FUNCTION_BLOCK "FB_CABINET_7P7-R24"
TITLE =Control cabinet 7P7-R24
{ S7_language := '9(1) Angielski (Stany Zjednoczone)  11.01.2022  09:45:15' }
VERSION : 0.1


VAR
  SM : STRUCT
   GeneralError : BOOL ;
   GeneralWarning : BOOL ;
   CtrlVoltageON : BOOL ;
   Auto : BOOL ;
   Manual : BOOL ;
   Local : BOOL ;
   Remote : BOOL ;
   CtrlRelease : BOOL ;
   CtrlRelease_A : BOOL ;
   res11 : BOOL ;
   res12 : BOOL ;
   res13 : BOOL ;
   res14 : BOOL ;
   res15 : BOOL ;
   LackCooling : BOOL ;
   LackHeating : BOOL ;
  END_STRUCT ;
  FM : STRUCT
   EnergyCounterFuse : BOOL ;
   ControlVoltage230VAC : BOOL ;
   ControlVoltage24VDC : BOOL ;
   ControlVoltage230VAC_MS : BOOL ;
   CabinetCoolingFuse : BOOL ;
   ProfiNetSwitchFault : BOOL ;
   MainSwitchFault : BOOL ;
   ExcessTemperature : BOOL ;
   ESTOP : BOOL ;
   FireAlarmPreWarning : BOOL ;
   FireAlarm : BOOL ;
   res13 : BOOL ;
   res14 : BOOL ;
   res15 : BOOL ;
   res16 : BOOL ;
   res17 : BOOL ;
  END_STRUCT ;
  CTRL : STRUCT
   ResetFault : BOOL ;
   ResetESTOP : BOOL ;
   LampTest : BOOL ;
   AutoStart : BOOL ;
   AutoStop : BOOL ;
   res05 : BOOL ;
   res06 : BOOL ;
   res07 : BOOL ;
   res10 : BOOL ;
   res11 : BOOL ;
   res12 : BOOL ;
   res13 : BOOL ;
   res14 : BOOL ;
   res15 : BOOL ;
   res16 : BOOL ;
   res17 : BOOL ;
  END_STRUCT ;
  CTRL_HMI : STRUCT
   ResetFault : BOOL ;
   Auto : BOOL ;
   Manual : BOOL ;
   res03 : BOOL ;
   res04 : BOOL ;
   res05 : BOOL ;
   res06 : BOOL ;
   res07 : BOOL ;
   ProductionOn : BOOL ;
   ProductionBreak : BOOL ;
   PlantOn : BOOL ;
   PlantOff : BOOL ;
   res14 : BOOL ;
   res15 : BOOL ;
   LackCooling : BOOL ;
   LackHeating : BOOL ;
  END_STRUCT ;
  EC : "UDT_EC";	//Energy Counter
END_VAR
VAR_TEMP
  ERROR_REL : BOOL ;
END_VAR
BEGIN
NETWORK
TITLE =STATUS



NETWORK
TITLE =CONTROL VOLTAGE ON
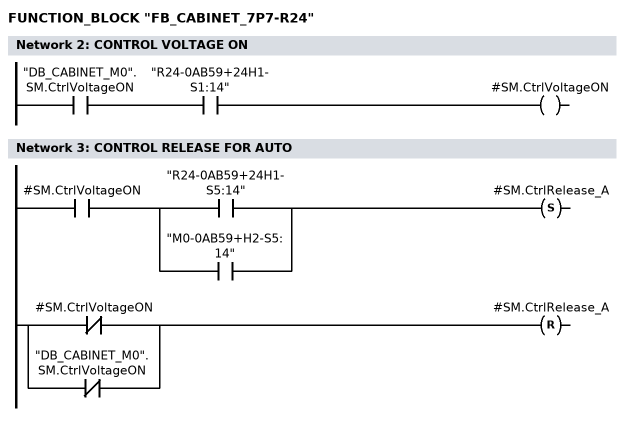
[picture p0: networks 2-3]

      U     "DB_CABINET_M0".SM.CtrlVoltageON;
      U     "R24-0AB59+24H1-S1:14";
      =     #SM.CtrlVoltageON;
NETWORK
TITLE =CONTROL RELEASE FOR AUTO

      U     #SM.CtrlVoltageON;
      U(    ;
      O     "R24-0AB59+24H1-S5:14";
      O     "M0-0AB59+H2-S5:14";
      )     ;
      S     #SM.CtrlRelease_A;
      U(    ;
      ON    #SM.CtrlVoltageON;
      ON    "DB_CABINET_M0".SM.CtrlVoltageON;
      )     ;
      R     #SM.CtrlRelease_A;
      NOP   0;
NETWORK
TITLE =AUTO/MANUAL MODE

      U(    ;
      U     "R24-0AB59+24H1-S2:14";
      S     #SM.Auto;
      U     "R24-0AB59+24H1-S2:22";
      R     #SM.Auto;
      U     #SM.Auto;
      )     ;
      NOT   ;
      =     #SM.Manual;
NETWORK
TITLE =LOCAL/REMOTE MODE

      U(    ;
      U     "DB_CABINET_M0".SM.Remote;
      S     #SM.Remote;
      U     "DB_CABINET_M0".SM.Local;
      R     #SM.Remote;
      U     #SM.Remote;
      )     ;
      NOT   ;
      =     #SM.Local;
NETWORK
TITLE =CONTROL RELEASE FROM CABINET
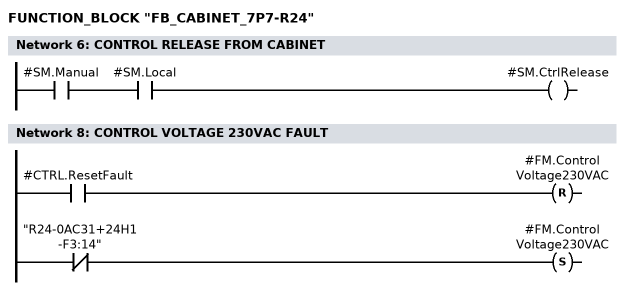
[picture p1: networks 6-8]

      U     #SM.Manual;
      U     #SM.Local;
      =     #SM.CtrlRelease;
NETWORK
TITLE =FAULTS



NETWORK
TITLE =CONTROL VOLTAGE 230VAC FAULT

      U     #CTRL.ResetFault;
      R     #FM.ControlVoltage230VAC;
      UN    "R24-0AC31+24H1-F3:14";
      S     #FM.ControlVoltage230VAC;
      NOP   0;
NETWORK
TITLE =CONTROL VOLTAGE 24V DC FAULT

      U     #CTRL.ResetFault;
      R     #FM.ControlVoltage24VDC;
      U(    ;
      O(    ;
      UN    "R24-0DC43+24H1-F1:7";
      L     S5T#300MS;
      SE    "T_R24-0DC43+24H1-F1";
      NOP   0;
      NOP   0;
      NOP   0;
      U     "T_R24-0DC43+24H1-F1";
      )     ;
      O(    ;
      UN    "R24-0DC43+24H1-F2:7";
      L     S5T#300MS;
      SE    "T_R24-0DC43+24H1-F2";
      NOP   0;
      NOP   0;
      NOP   0;
      U     "T_R24-0DC43+24H1-F2";
      )     ;
      )     ;
      S     #FM.ControlVoltage24VDC;
      NOP   0;
NETWORK
TITLE =CONTROL VOLTAGE 230V AC BEFORE MAIN SWITCH FAULT
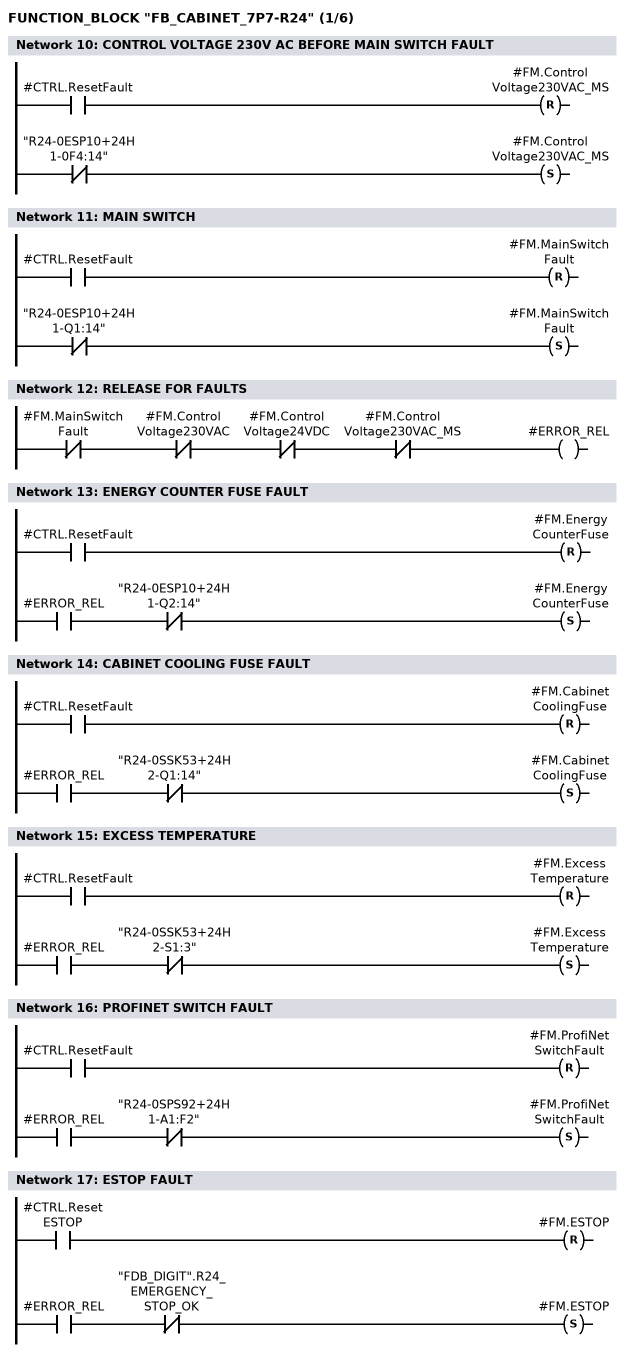
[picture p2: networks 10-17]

      U     #CTRL.ResetFault;
      R     #FM.ControlVoltage230VAC_MS;
      UN    "R24-0ESP10+24H1-0F4:14";
      S     #FM.ControlVoltage230VAC_MS;
      NOP   0;
NETWORK
TITLE =MAIN SWITCH

      U     #CTRL.ResetFault;
      R     #FM.MainSwitchFault;
      UN    "R24-0ESP10+24H1-Q1:14";
      S     #FM.MainSwitchFault;
      NOP   0;
NETWORK
TITLE =RELEASE FOR FAULTS

      UN    #FM.MainSwitchFault;
      UN    #FM.ControlVoltage230VAC;
      UN    #FM.ControlVoltage24VDC;
      UN    #FM.ControlVoltage230VAC_MS;
      =     #ERROR_REL;
NETWORK
TITLE =ENERGY COUNTER FUSE FAULT

      U     #CTRL.ResetFault;
      R     #FM.EnergyCounterFuse;
      U     #ERROR_REL;
      UN    "R24-0ESP10+24H1-Q2:14";
      S     #FM.EnergyCounterFuse;
      NOP   0;
NETWORK
TITLE =CABINET COOLING FUSE FAULT

      U     #CTRL.ResetFault;
      R     #FM.CabinetCoolingFuse;
      U     #ERROR_REL;
      UN    "R24-0SSK53+24H2-Q1:14";
      S     #FM.CabinetCoolingFuse;
      NOP   0;
NETWORK
TITLE =EXCESS TEMPERATURE

      U     #CTRL.ResetFault;
      R     #FM.ExcessTemperature;
      U     #ERROR_REL;
      UN    "R24-0SSK53+24H2-S1:3";
      S     #FM.ExcessTemperature;
      NOP   0;
NETWORK
TITLE =PROFINET SWITCH FAULT

      U     #CTRL.ResetFault;
      R     #FM.ProfiNetSwitchFault;
      U     #ERROR_REL;
      UN    "R24-0SPS92+24H1-A1:F2";
      S     #FM.ProfiNetSwitchFault;
      NOP   0;
NETWORK
TITLE =ESTOP FAULT

      U     #CTRL.ResetESTOP;
      R     #FM.ESTOP;
      U     #ERROR_REL;
      UN    "FDB_DIGIT".R24_EMERGENCY_STOP_OK;
      S     #FM.ESTOP;
      NOP   0;
NETWORK
TITLE =ESTOP CONTROL CABINET OK
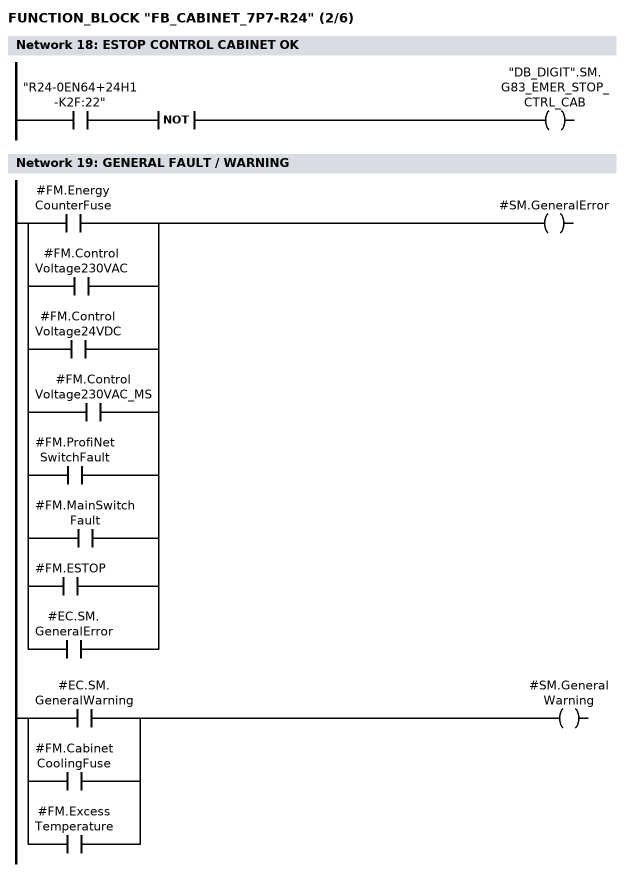
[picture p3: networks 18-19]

      U     "R24-0EN64+24H1-K2F:22";
      NOT   ;
      =     "DB_DIGIT".SM.G83_EMER_STOP_CTRL_CAB;
NETWORK
TITLE =GENERAL FAULT / WARNING


      U     #FM.EnergyCounterFuse;
      O     #FM.ControlVoltage230VAC;
      O     #FM.ControlVoltage24VDC;
      O     #FM.ControlVoltage230VAC_MS;
      O     #FM.ProfiNetSwitchFault;
      O     #FM.MainSwitchFault;
      O     #FM.ESTOP;
      O     #EC.SM.GeneralError;
      =     #SM.GeneralError;



      U     #EC.SM.GeneralWarning;
      O     #FM.CabinetCoolingFuse;
      O     #FM.ExcessTemperature;
      =     #SM.GeneralWarning;

NETWORK
TITLE =CONTROL SIGNALS



NETWORK
TITLE =RESET FAULT
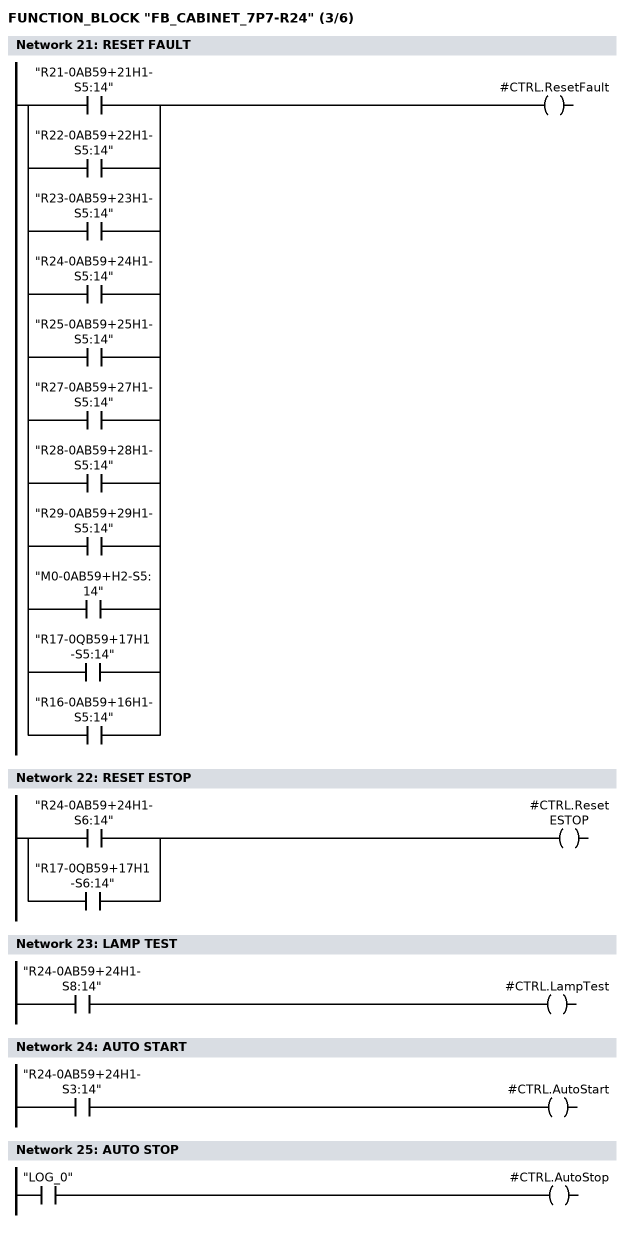
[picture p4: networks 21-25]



      O     "R21-0AB59+21H1-S5:14";
      O     "R22-0AB59+22H1-S5:14";
      O     "R23-0AB59+23H1-S5:14";
      O     "R24-0AB59+24H1-S5:14";
      O     "R25-0AB59+25H1-S5:14";
      O     "R27-0AB59+27H1-S5:14";
      O     "R28-0AB59+28H1-S5:14";
      O     "R29-0AB59+29H1-S5:14";
      O     "M0-0AB59+H2-S5:14";
      O     "R17-0QB59+17H1-S5:14";
      O     "R16-0AB59+16H1-S5:14";
      =     #CTRL.ResetFault;
NETWORK
TITLE =RESET ESTOP



      O     "R24-0AB59+24H1-S6:14";
      O     "R17-0QB59+17H1-S6:14";
      =     #CTRL.ResetESTOP;
NETWORK
TITLE =LAMP TEST



      U     "R24-0AB59+24H1-S8:14";
      =     #CTRL.LampTest;
NETWORK
TITLE =AUTO START



      U     "R24-0AB59+24H1-S3:14";
      =     #CTRL.AutoStart;
NETWORK
TITLE =AUTO STOP



      U     "LOG_0";
      =     #CTRL.AutoStop;
NETWORK
TITLE =BUTTON LAMPS
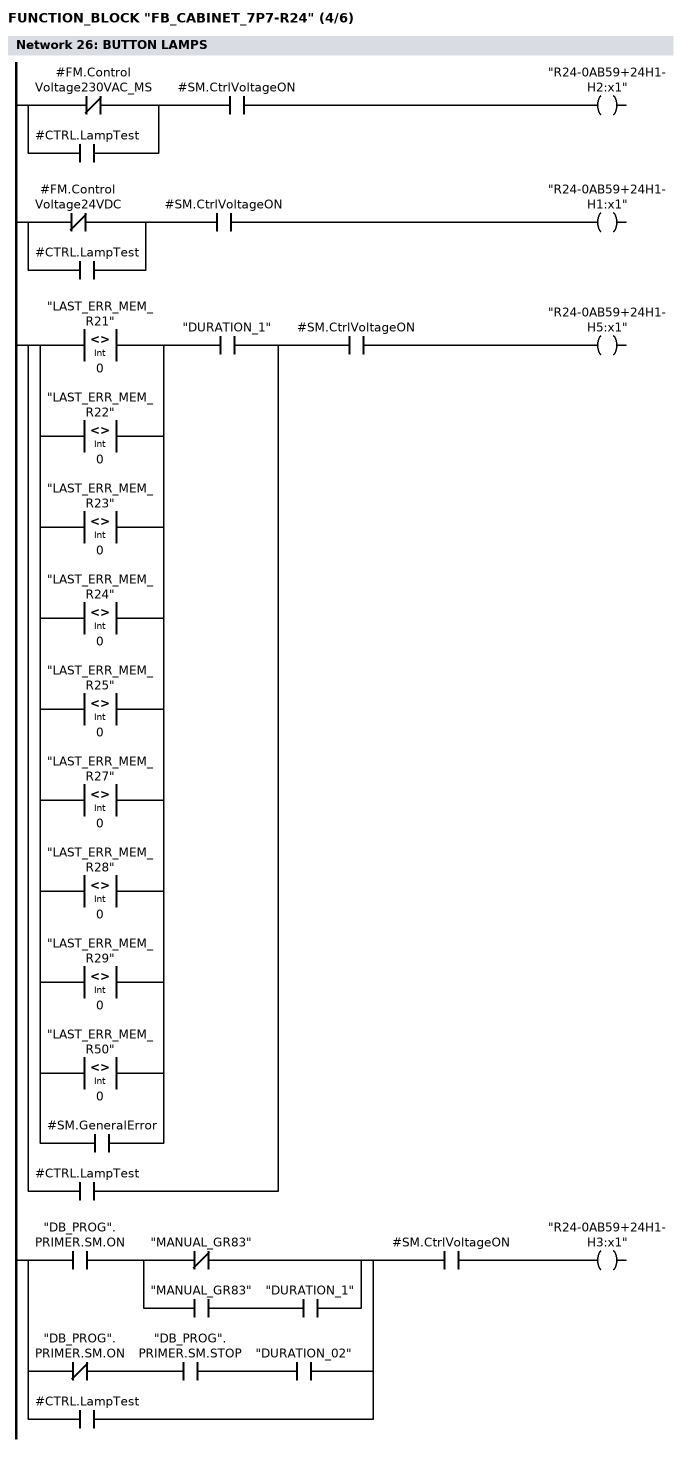
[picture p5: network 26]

// CONTROL VOLTAGE 230V AC
      U(    ;
      ON    #FM.ControlVoltage230VAC_MS;
      O     #CTRL.LampTest;
      )     ;
      U     #SM.CtrlVoltageON;
      =     "R24-0AB59+24H1-H2:x1";

// CONTROL VOLTAGE 24V DC
      U(    ;
      ON    #FM.ControlVoltage24VDC;
      O     #CTRL.LampTest;
      )     ;
      U     #SM.CtrlVoltageON;
      =     "R24-0AB59+24H1-H1:x1";

// RESET
      U(    ;
      L     "LAST_ERR_MEM_R21";
      L     0;
      <>I   ;
      )     ;
      O(    ;
      L     "LAST_ERR_MEM_R22";
      L     0;
      <>I   ;
      )     ;
      O(    ;
      L     "LAST_ERR_MEM_R23";
      L     0;
      <>I   ;
      )     ;
      O(    ;
      L     "LAST_ERR_MEM_R24";
      L     0;
      <>I   ;
      )     ;
      O(    ;
      L     "LAST_ERR_MEM_R25";
      L     0;
      <>I   ;
      )     ;
      O(    ;
      L     "LAST_ERR_MEM_R27";
      L     0;
      <>I   ;
      )     ;
      O(    ;
      L     "LAST_ERR_MEM_R28";
      L     0;
      <>I   ;
      )     ;
      O(    ;
      L     "LAST_ERR_MEM_R29";
      L     0;
      <>I   ;
      )     ;
      O(    ;
      L     "LAST_ERR_MEM_R50";
      L     0;
      <>I   ;
      )     ;
      O     #SM.GeneralError;
      U     "DURATION_1";
      O     #CTRL.LampTest;
      U     #SM.CtrlVoltageON;
      =     "R24-0AB59+24H1-H5:x1";

// AUTOMATIC START
      U(    ;
      U     "DB_PROG".PRIMER.SM.ON;
      U(    ;
      ON    "MANUAL_GR83";
      O     ;
      U     "MANUAL_GR83";
      U     "DURATION_1";
      )     ;
      O     ;
      UN    "DB_PROG".PRIMER.SM.ON;
      U     "DB_PROG".PRIMER.SM.STOP;
      U     "DURATION_02";
      O     #CTRL.LampTest;
      )     ;
      U     #SM.CtrlVoltageON;

      =     "R24-0AB59+24H1-H3:x1";
NETWORK
TITLE =LIGHT TOWER
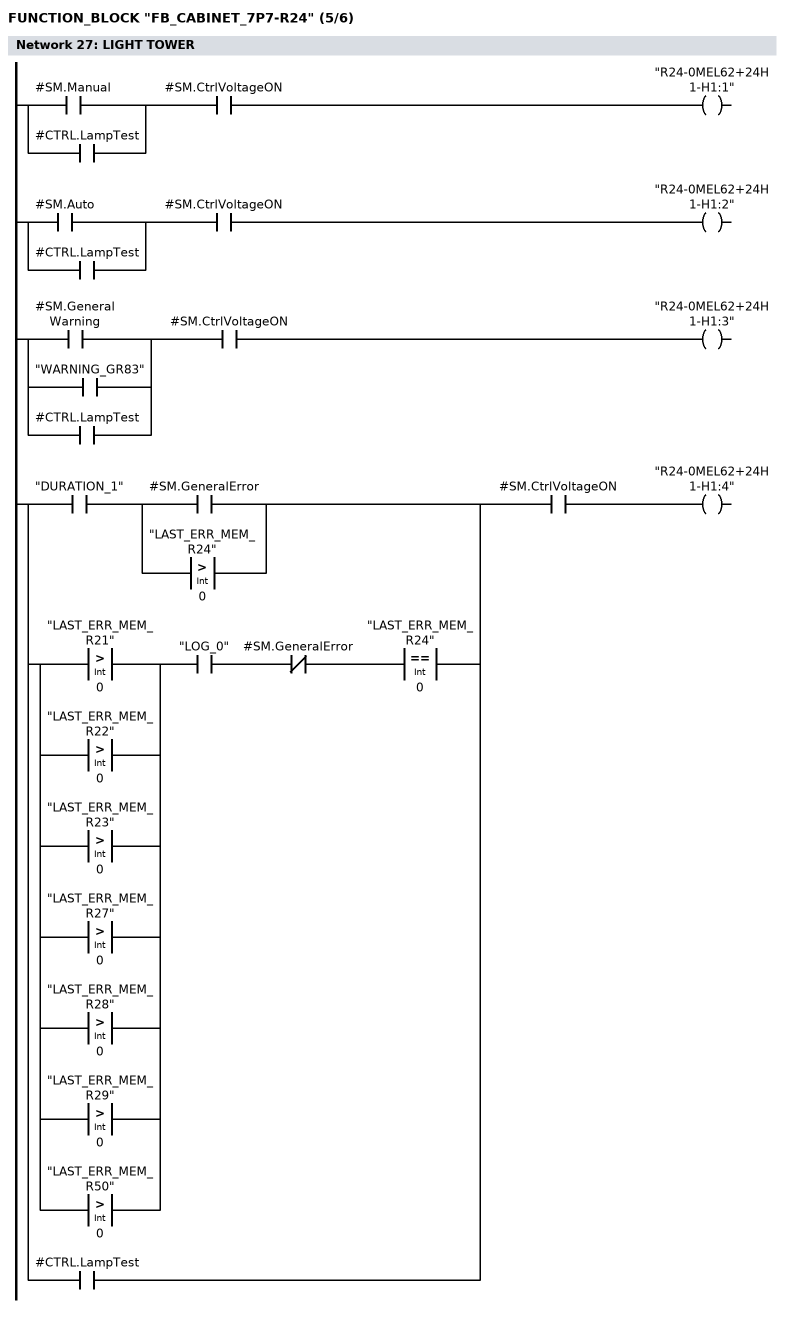
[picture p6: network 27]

// MANUAL
      U(    ;
      O     #SM.Manual;
      O     #CTRL.LampTest;
      )     ;
      U     #SM.CtrlVoltageON;
      =     "R24-0MEL62+24H1-H1:1";

// AUTO
      U(    ;
      O     #SM.Auto;
      O     #CTRL.LampTest;
      )     ;
      U     #SM.CtrlVoltageON;
      =     "R24-0MEL62+24H1-H1:2";

// WARNING
      U(    ;
      O     #SM.GeneralWarning;
      O     "WARNING_GR83";
      O     #CTRL.LampTest;
      )     ;
      U     #SM.CtrlVoltageON;
      =     "R24-0MEL62+24H1-H1:3";

// FAULT
      U(    ;
      U     "DURATION_1";
      U(    ;
      O     #SM.GeneralError;
      O(    ;
      L     "LAST_ERR_MEM_R24";
      L     0;
      >I    ;
      )     ;
      )     ;
      O     ;
      U(    ;
      O(    ;
      L     "LAST_ERR_MEM_R21";
      L     0;
      >I    ;
      )     ;
      O(    ;
      L     "LAST_ERR_MEM_R22";
      L     0;
      >I    ;
      )     ;
      O(    ;
      L     "LAST_ERR_MEM_R23";
      L     0;
      >I    ;
      )     ;
      O(    ;
      L     "LAST_ERR_MEM_R27";
      L     0;
      >I    ;
      )     ;
      O(    ;
      L     "LAST_ERR_MEM_R28";
      L     0;
      >I    ;
      )     ;
      O(    ;
      L     "LAST_ERR_MEM_R29";
      L     0;
      >I    ;
      )     ;
      O(    ;
      L     "LAST_ERR_MEM_R50";
      L     0;
      >I    ;
      )     ;
      )     ;
      U     "LOG_0";
      UN    #SM.GeneralError;
      U(    ;
      L     "LAST_ERR_MEM_R24";
      L     0;
      ==I   ;
      )     ;
      O     #CTRL.LampTest;
      )     ;
      U     #SM.CtrlVoltageON;
      =     "R24-0MEL62+24H1-H1:4";
NETWORK
TITLE =HORN
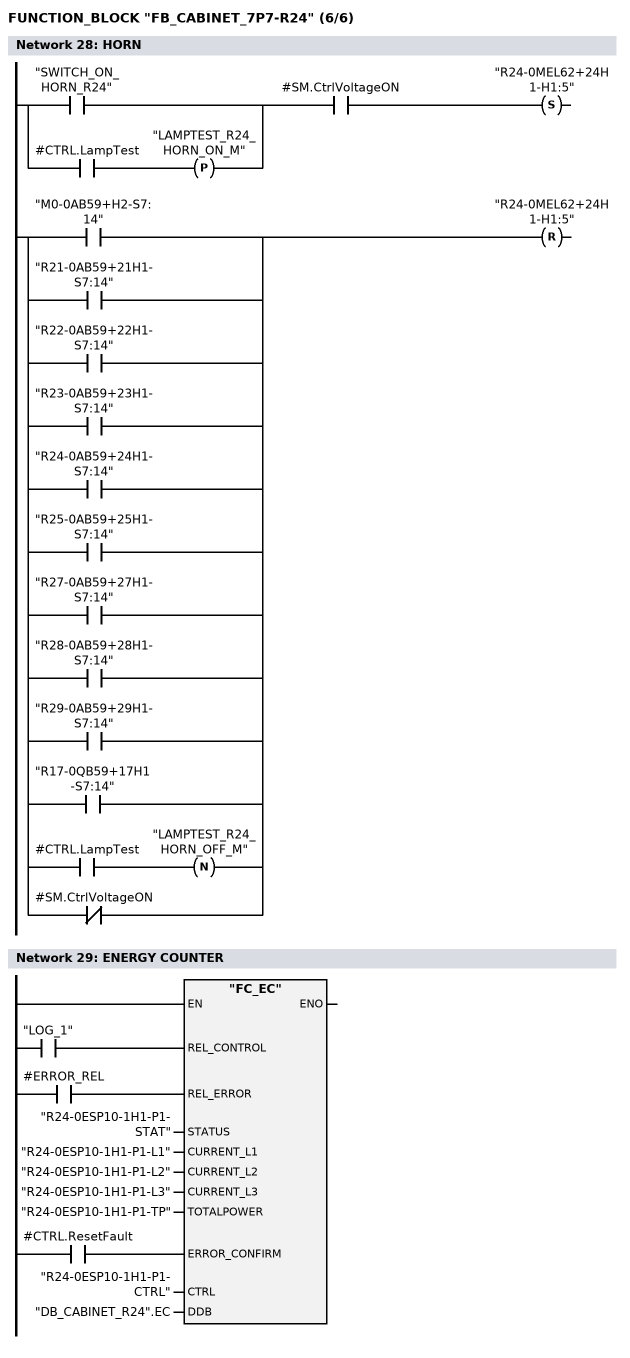
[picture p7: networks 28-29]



      U(    ;
      O     "SWITCH_ON_HORN_R24";
      O(    ;
      U     #CTRL.LampTest;
      FP    "LAMPTEST_R24_HORN_ON_M";
      )     ;
      )     ;
      U     #SM.CtrlVoltageON;
      S     "R24-0MEL62+24H1-H1:5";
      U(    ;
      O     "M0-0AB59+H2-S7:14";
      O     "R21-0AB59+21H1-S7:14";
      O     "R22-0AB59+22H1-S7:14";
      O     "R23-0AB59+23H1-S7:14";
      O     "R24-0AB59+24H1-S7:14";
      O     "R25-0AB59+25H1-S7:14";
      O     "R27-0AB59+27H1-S7:14";
      O     "R28-0AB59+28H1-S7:14";
      O     "R29-0AB59+29H1-S7:14";
      O     "R17-0QB59+17H1-S7:14";
      O(    ;
      U     #CTRL.LampTest;
      FN    "LAMPTEST_R24_HORN_OFF_M";
      )     ;
      ON    #SM.CtrlVoltageON;
      )     ;
      R     "R24-0MEL62+24H1-H1:5";
      NOP   0;
NETWORK
TITLE =ENERGY COUNTER

      U     "LOG_1";
      =     L      1.0;
      BLD   103;
      U     #ERROR_REL;
      =     L      1.1;
      BLD   103;
      U     #CTRL.ResetFault;
      =     L      1.2;
      BLD   103;
      CALL "FC_EC" (
           REL_CONTROL              := L      1.0,
           REL_ERROR                := L      1.1,
           STATUS                   := "R24-0ESP10-1H1-P1-STAT",
           CURRENT_L1               := "R24-0ESP10-1H1-P1-L1",
           CURRENT_L2               := "R24-0ESP10-1H1-P1-L2",
           CURRENT_L3               := "R24-0ESP10-1H1-P1-L3",
           TOTALPOWER               := "R24-0ESP10-1H1-P1-TP",
           ERROR_CONFIRM            := L      1.2,
           CTRL                     := "R24-0ESP10-1H1-P1-CTRL",
           DDB                      := "DB_CABINET_R24".EC);
      NOP   0;
NETWORK
TITLE =END

END_FUNCTION_BLOCK

